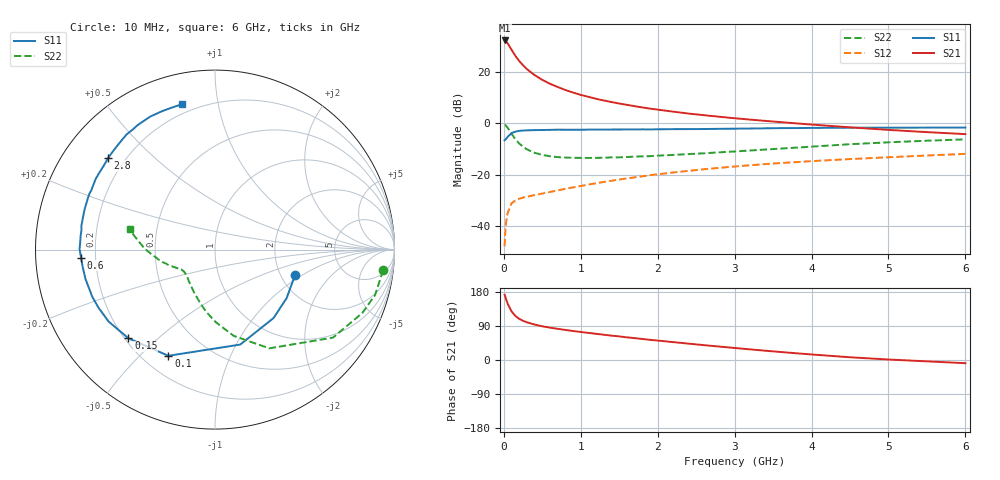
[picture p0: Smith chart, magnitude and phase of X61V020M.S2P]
! SIEMENS Small Signal Semiconductors
! BFP193W
! Si NPN RF Bipolar Junction Transistor in SOT343
! VCE = 1 V  IC = 20 mA
! Common Emitter S-Parameters:  April 1994
# GHz  S  MA  R  50
!  f  S11  S21  S12  S22
! GHz  MAG  ANG  MAG  ANG  MAG  ANG  MAG  ANG
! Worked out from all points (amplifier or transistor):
!   40 points, 10 MHz to 6 GHz, reference 50 ohm
!   highest |S21| = 32.4 dB at 10 MHz (marker M1)
!   |S21| within 3 dB of that: start of sweep to 87.3 MHz
!   unconditionally stable (mu >= 1): 843.1 MHz to 5.568 GHz
!   at 200 MHz: K = 0.37, MSG = 26.9 dB, |S12| = -29.4 dB
!   at 1.5 GHz: K = 1.15, MAG = 12.5 dB, |S12| = -21.9 dB
!   at 6 GHz: K = 0.98, MSG = 3.9 dB, |S12| = -11.9 dB
!   S11 on the Smith chart (normalised r, x): 10 MHz: 2.39, -0.86; 100 MHz: 0.30, -0.61; 150 MHz: 0.21, -0.40; 600 MHz: 0.14, -0.03; 2.8 GHz: 0.14, +0.36; 6 GHz: 0.15, +0.79
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0.01  0.4681 -17.5  41.73 172.4  0.004 83.4  0.9439 -7.0
0.02  0.4822 -34.2  41.13 166.4  0.0083 77.5  0.9271 -15.8
0.03  0.5017 -49.4  40.01 160.0  0.0118 72.9  0.8941 -23.2
0.05  0.5474 -75.1  36.49 148.4  0.0179 62.3  0.8201 -36.7
0.1  0.6461 -113.7  27.5 128.4  0.0273 47.3  0.6278 -61.2
0.15  0.6905 -134.3  20.9 116.1  0.0314 39.8  0.4915 -77.8
0.2  0.7155 -145.9  16.54 108.7  0.0337 36.6  0.4053 -89.2
0.25  0.7253 -153.5  13.66 103.4  0.0356 35.4  0.3511 -97.9
0.3  0.7326 -159.0  11.49 99.5  0.0371 35.7  0.3109 -105.1
0.4  0.7399 -167.2  8.782 93.5  0.0397 36.9  0.2669 -115.7
0.5  0.7435 -172.5  7.103 89.0  0.0427 39.1  0.2427 -123.5
0.6  0.7474 -176.6  5.943 85.3  0.0458 41.5  0.2284 -129.5
0.8  0.7521 177.0  4.497 79.3  0.0527 45.6  0.215 -137.2
1.1  0.7561 169.8  3.307 71.5  0.0639 49.4  0.2116 -144.3
1.3  0.7576 165.6  2.804 66.6  0.0719 51.1  0.2142 -146.9
1.6  0.7619 159.7  2.303 59.8  0.0844 52.4  0.2204 -150.0
2.2  0.7728 149.3  1.699 47.2  0.1099 52.0  0.2423 -155.9
2.8  0.7841 139.4  1.35 35.5  0.1355 49.7  0.2724 -161.4
3.2  0.7946 133.3  1.188 28.1  0.1521 47.3  0.2958 -165.9
4.5  0.8243 116.0  0.838 7.2  0.201 38.8  0.3924 179.1
5.5  0.8268 107.1  0.676 -3.6  0.236 32.4  0.459 170.0
6  0.8307 102.8  0.618 -8.4  0.2541 29.6  0.4887 166.4
